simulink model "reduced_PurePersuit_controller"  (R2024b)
settings: Solver=ode1be  StartTime=0.0  StopTime=100  FixedStep=0.01  RelTol=1e-3
undefined symbols (not defined in the file): opti_ref_values, startPose, StepSize, VehicleParams
libraries: slpidlib x1, robotalgslib x1

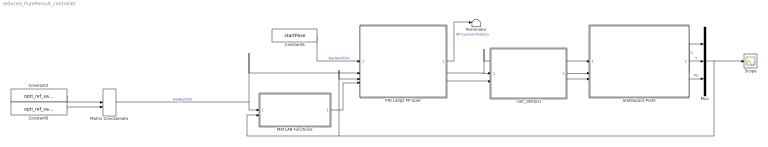
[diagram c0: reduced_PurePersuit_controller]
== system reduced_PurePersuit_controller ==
  Constant2 : Constant  Value=opti_ref_values(:, 1)
  Constant5 : Constant  Value=startPose
  Constant6 : Constant  Value=opti_ref_values(:, 2)
  MATLAB Function2 : MATLAB Function  TreatAsAtomicUnit=on
  Matrix Concatenate : Concatenate  Mode=Multidimensional array  ConcatenateDimension=2
  Mux : Mux  Inputs=3
  PID Längs PP Quer : Subsystem
  Scope : Scope
  StateSpace Plant : Subsystem
  Terminator : Terminator
  calc_delta(s) : Subsystem
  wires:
  Matrix Concatenate/1 -> PID Längs PP Quer/2(Waypoints (HybridAStar)), MATLAB Function2/1(Ref)  "wegpunkte"
  Constant2/1 -> Matrix Concatenate/1
  Constant6/1 -> Matrix Concatenate/2
  Constant5/1 -> PID Längs PP Quer/1(Start Position)  "startposition"
  MATLAB Function2/1(e_long) -> PID Längs PP Quer/4(e_long)
  PID Längs PP Quer/2(v_vehicleBody) -> StateSpace Plant/1(v_vehicleBody), calc_delta(s)/1(vx)
  PID Längs PP Quer/3(Psi_dot) -> calc_delta(s)/2(psi_dot)
  PID Längs PP Quer/1(PP Current Position) -> Terminator/1  "PP Current Position"
  calc_delta(s)/1(delta_f) -> StateSpace Plant/2(Delta_F)
  calc_delta(s)/2(delta_r) -> StateSpace Plant/3(Delta_R)
  StateSpace Plant/1(X) -> Mux/1  "X"
  StateSpace Plant/2(Y) -> Mux/2  "Y"
  StateSpace Plant/3(psi) -> Mux/3  "Psi"
  Mux/1 -> PID Längs PP Quer/3(Current Position), MATLAB Function2/2(Act), Scope/1

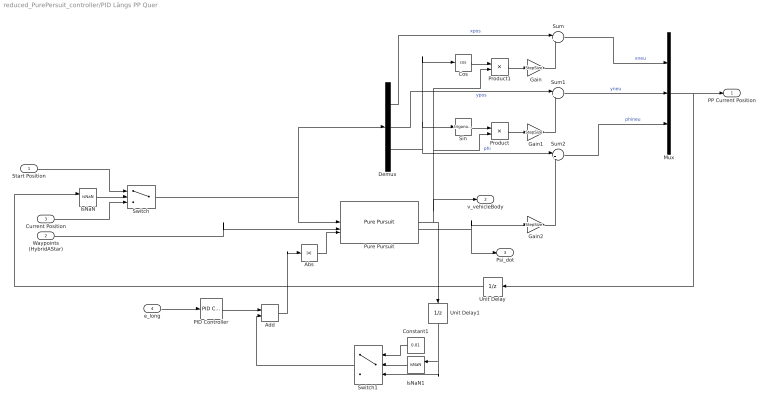
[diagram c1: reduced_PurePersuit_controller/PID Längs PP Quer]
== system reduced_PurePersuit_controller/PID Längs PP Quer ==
  Start Position : Inport
  Waypoints (HybridAStar) : Inport  Port=2
  Current Position : Inport  Port=3
  e_long : Inport  Port=4
  Abs : Abs
  Add : Sum
  Constant1 : Constant  Value=0.01
  Cos : Trigonometry  Operator=cos
  Demux : Demux  Outputs=3
  Gain : Gain  Gain=StepSize
  Gain1 : Gain  Gain=StepSize
  Gain2 : Gain  Gain=StepSize
  IsNaN : RelationalOperator  Operator=isNaN  OutDataTypeStr=boolean  RndMeth=Simplest
  IsNaN1 : RelationalOperator  Operator=isNaN  OutDataTypeStr=boolean  RndMeth=Simplest
  Mux : Mux  Inputs=3
  PID Controller : slpidlib/PID Controller  Controller=PID  Form=Parallel  TimeDomain=Continuous-time  UseExternalTs=off  SampleTime=-1  IntegratorMethod=Forward Euler  FilterMethod=Forward Euler  ControllerParametersSource=internal  P=0.4  I=0  UseKiTs=off  D=0  UseExternalDerivativeSource=off  N=100  UseFilter=on  TunerSelectOption=Transfer Function Based (PID Tuner App)  InitialConditionSource=internal  InitialConditionForIntegrator=0  InitialConditionForFilter=0  DifferentiatorICPrevScaledInput=0  ExternalReset=none  TrackingMode=off  Kt=1  LimitOutput=on  SatLimitsSource=internal  UpperSaturationLimit=1  LowerSaturationLimit=-1  LinearizeAsGain=on  AntiWindupMode=clamping  Kb=1  LimitIntegrator=off  UpperIntegratorSaturationLimit=inf  LowerIntegratorSaturationLimit=-inf  POutMin=[]  POutMax=[]  IOutMin=[]  IOutMax=[]  DOutMin=[]  DOutMax=[]  NOutMin=[]  NOutMax=[]  SumOutMin=[]  SumOutMax=[]  SaturationOutMin=[]  SaturationOutMax=[]  PParamMin=[]  PParamMax=[]  IParamMin=[]  IParamMax=[]  DParamMin=[]  DParamMax=[]  NParamMin=[]  NParamMax=[]  KbParamMin=[]  KbParamMax=[]  KtParamMin=[]  KtParamMax=[]  KbOutMin=[]  KbOutMax=[]  KtOutMin=[]  KtOutMax=[]  IntegratorOutMin=[]  IntegratorOutMax=[]  FilterOutMin=[]  FilterOutMax=[]  SumI1OutMin=[]  SumI1OutMax=[]  SumI2OutMin=[]  SumI2OutMax=[]  SumI3OutMin=[]  SumI3OutMax=[]  SumI4OutMin=[]  SumI4OutMax=[]  SumDOutMin=[]  SumDOutMax=[]  DifferentiatorOutMin=[]  DifferentiatorOutMax=[]  FilterDiffOutCoefMin=[]  FilterDiffOutCoefMax=[]  ReciprocalOutMin=[]  ReciprocalOutMax=[]  SumDenOutMin=[]  SumDenOutMax=[]  SumNumOutMin=[]  SumNumOutMax=[]  DivideOutMin=[]  DivideOutMax=[]  UdiffTsProdOutMin=[]  UdiffTsProdOutMax=[]  NTsProdOutMin=[]  NTsProdOutMax=[]  UintegralTsProdOutMin=[]  UintegralTsProdOutMax=[]  UngainTsProdOutMin=[]  UngainTsProdOutMax=[]  ClampingZeroOutDataTypeStr=Inherit: Inherit via back propagation  ClampingZeroOutMin=[]  ClampingZeroOutMax=[]  FilterDenConstantOutDataTypeStr=Inherit: Inherit via back propagation  FilterDenConstantOutMin=[]  FilterDenConstantOutMax=[]  PCopyOutDataTypeStr=Inherit: Inherit via back propagation  PCopyOutMin=[]  PCopyOutMax=[]  NCopyOutDataTypeStr=Inherit: Inherit via back propagation  NCopyOutMin=[]  NCopyOutMax=[]  IntegratorContinuousStateAttributes=''  IntegratorStateMustResolveToSignalObject=off  IntegratorRTWStateStorageClass=Auto  FilterContinuousStateAttributes=''  FilterStateMustResolveToSignalObject=off  FilterRTWStateStorageClass=Auto  ParallelPVariant=InternalParameters  IdealPVariant=Disabled  IVariant=InternalParameters  DVariant=InternalParameters  IntegratorVariant=Continuous  SatVariant=Enabled  AWVariant=ContClampingParallel  PCopyVariant=Disabled  TRVariant=Disabled  FdbkBlocksVariant=Forward  IdealPFdbkVariant=Disabled  SatFdbkVariant=Disabled  DerivativeFilterVariant=ContFilter  NVariant=InternalParameters  NCopyVariant=Disabled  FilterICVariant=InternalICsFilter  IntegratorICVariant=InternalICs  ExternalResetVariant=Disabled  TRSumVariant=Passthrough  SumFdbkVariant=Disabled  SumVariant=Sum_PID  TsampFilterVariant=InternalTs  TsampNgainVariant=Passthrough  TsampIntegralVariant=Disabled_SignalSpec  ExternalSaturationOutDataTypeStr=Inherit: Same as second input  DerivativeSourceVariant=ErrorSignal  PreIntVariant=InternalPreInt
  Product : Product
  Product1 : Product
  Pure Pursuit : robotalgslib/Pure Pursuit  DesiredLinearVelocityPort=on  DesiredLinearVelocity=v_vb  MaxAngularVelocity=psi_dot_max  LookaheadDistancePort=off  LookaheadDistance=lookahead_distance  TargetDirPort=off  SimulateUsing=Code generation
  Sin : Trigonometry
  Sum : Sum  Inputs=|++
  Sum1 : Sum  Inputs=|++
  Sum2 : Sum  Inputs=|++
  Switch : Switch  Criteria=u2 ~= 0
  Switch1 : Switch  Criteria=u2 ~= 0
  Unit Delay : UnitDelay  SampleTime=-1  HasFrameUpgradeWarning=on
  Unit Delay1 : UnitDelay  SampleTime=-1  HasFrameUpgradeWarning=on
  PP Current Position : Outport
  v_vehicleBody : Outport  Port=2
  Psi_dot : Outport  Port=3
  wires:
  Unit Delay/1 -> IsNaN/1
  Sum/1 -> Mux/1  "xneu"
  Demux/1 -> Sum/1  "xpos"
  Waypoints (HybridAStar)/1 -> Pure Pursuit/2
  Cos/1 -> Product1/1
  Gain2/1 -> Sum2/2
  Pure Pursuit/2 -> Psi_dot/1, Gain2/1
  Gain/1 -> Sum/2
  Sum2/1 -> Mux/3  "phineu"
  Demux/2 -> Sum1/1  "ypos"
  Sin/1 -> Product/1
  Mux/1 -> Unit Delay/1, PP Current Position/1
  Gain1/1 -> Sum1/2
  Product/1 -> Gain1/1
  Sum1/1 -> Mux/2  "yneu"
  IsNaN/1 -> Switch/2
  Start Position/1 -> Switch/1
  Switch/1 -> Demux/1, Pure Pursuit/1
  Demux/3 -> Sum2/1, Sin/1, Cos/1  "phi"
  Product1/1 -> Gain/1
  Current Position/1 -> Switch/3
  Constant1/1 -> Switch1/1
  IsNaN1/1 -> Switch1/2
  Switch1/1 -> Add/2
  e_long/1 -> PID Controller/1
  PID Controller/1 -> Add/1
  Add/1 -> Abs/1
  Pure Pursuit/1 -> Unit Delay1/1, Product/2, Product1/2, v_vehicleBody/1
  Abs/1 -> Pure Pursuit/3
  Unit Delay1/1 -> Switch1/3, IsNaN1/1

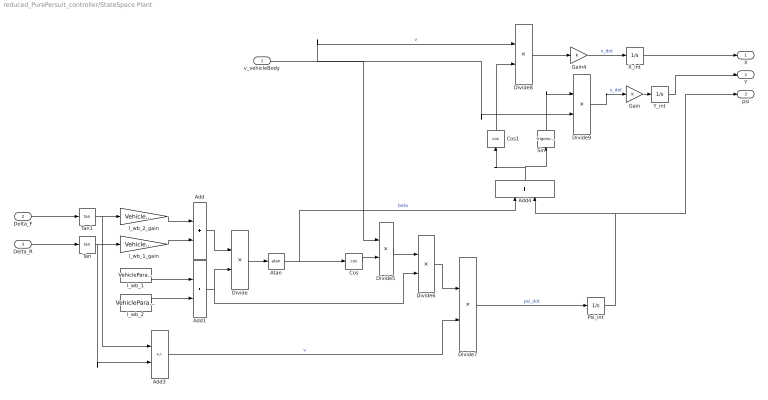
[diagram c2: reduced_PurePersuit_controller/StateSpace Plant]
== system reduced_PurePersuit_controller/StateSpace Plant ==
  v_vehicleBody : Inport
  Delta_F : Inport  Port=2
  Delta_R : Inport  Port=3
  Add : Sum
  Add1 : Sum
  Add3 : Sum  Inputs=+-
  Add4 : Sum
  Atan : Trigonometry  Operator=atan
  Cos : Trigonometry  Operator=cos
  Cos1 : Trigonometry  Operator=cos
  Divide : Product  Inputs=*/
  Divide{5,7..9} (4 alike) : Product  Inputs=**
  Divide6 : Product  Inputs=*/
  Gain : Gain
  Gain4 : Gain
  Psi_int : Integrator
  Sin : Trigonometry
  Tan : Trigonometry  Operator=tan
  Tan1 : Trigonometry  Operator=tan
  X_int : Integrator
  Y_int : Integrator
  l_wb_1 : Constant  Value=VehicleParams.dim_Wheelbase_Road/2
  l_wb_1_gain : Gain  Gain=VehicleParams.dim_Wheelbase_Road/2
  l_wb_2 : Constant  Value=VehicleParams.dim_Wheelbase_Road/2
  l_wb_2_gain : Gain  Gain=VehicleParams.dim_Wheelbase_Road/2
  X : Outport
  Y : Outport  Port=2
  psi : Outport  Port=3
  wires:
  v_vehicleBody/1 -> Divide5/1, Divide9/2, Divide8/1  "v"
  Psi_int/1 -> psi/1, Add4/2
  Add4/1 -> Cos1/1, Sin/1
  Cos1/1 -> Divide8/2
  Sin/1 -> Divide9/1
  Divide8/1 -> Gain4/1
  Divide9/1 -> Gain/1  "y_dot"
  X_int/1 -> X/1
  Y_int/1 -> Y/1
  Gain4/1 -> X_int/1  "x_dot"
  Atan/1 -> Add4/1, Cos/1  "beta"
  Cos/1 -> Divide5/2
  Divide6/1 -> Divide7/1
  l_wb_1_gain/1 -> Add/2
  Add/1 -> Divide/1
  Divide7/1 -> Psi_int/1  "psi_dot"
  Add3/1 -> Divide7/2  "v"
  Add1/1 -> Divide6/2, Divide/2
  Divide5/1 -> Divide6/1
  l_wb_2/1 -> Add1/2
  Divide/1 -> Atan/1
  Tan1/1 -> Add3/1, l_wb_2_gain/1
  l_wb_1/1 -> Add1/1
  Tan/1 -> Add3/2, l_wb_1_gain/1
  l_wb_2_gain/1 -> Add/1
  Gain/1 -> Y_int/1
  Delta_F/1 -> Tan1/1
  Delta_R/1 -> Tan/1

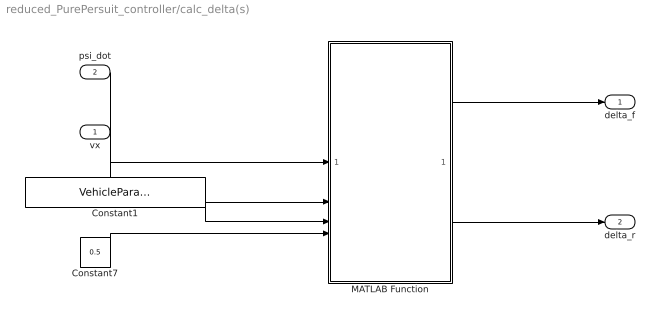
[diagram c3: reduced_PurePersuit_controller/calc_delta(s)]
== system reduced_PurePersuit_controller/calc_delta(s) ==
  vx : Inport
  psi_dot : Inport  Port=2
  Constant1 : Constant  Value=VehicleParams.dim_Wheelbase_Road
  Constant7 : Constant  Value=0.5
  MATLAB Function : MATLAB Function  TreatAsAtomicUnit=on
  delta_f : Outport
  delta_r : Outport  Port=2
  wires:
  vx/1 -> MATLAB Function/2(vx)
  Constant7/1 -> MATLAB Function/4(k)
  Constant1/1 -> MATLAB Function/3(L)
  psi_dot/1 -> MATLAB Function/1(psi_dot)
  MATLAB Function/1(delta_f) -> delta_f/1
  MATLAB Function/2(delta_r) -> delta_r/1

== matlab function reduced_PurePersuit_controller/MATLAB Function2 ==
function e_long = calculate_longitudinal_error(Ref, Act)
    % Berechnet den Längsfehler zwischen einem Referenzpfad und einer echten Position in Echtzeit.
    %
    % Inputs:
    %   X_ref, Y_ref, Psi_ref: Skalare Werte der Referenzposition und -orientierung
    %   X_act, Y_act: Skalare Werte der aktuellen Position
    %
    % Output:
    %   longitudinal_error: Skalarer Wert des berechneten Längsfehlers
    
    X_ref = Ref(1);
    Y_ref = Ref(2);
    Psi_ref = Ref(3);

    X_act = Act(1);
    Y_act = Act(2);
    Psi_act = Act(3);

    % Berechnet den Längsfehler zwischen dem aktuellen Fahrzeugpunkt und dem Referenzpunkt.
    %
    % Eingabe:
    %   X_ref, Y_ref  - Koordinaten des aktuellen Referenzpunktes
    %   Psi_ref       - Orientierung des Referenzpfads am aktuellen Punkt (in Radiant)
    %   X_act, Y_act  - Koordinaten des aktuellen Fahrzeugpunktes
    %
    % Ausgabe:
    %   e_long - Längsfehler (positiv: vor dem Referenzpunkt, negativ: dahinter)

    % Vektor vom Referenzpunkt zum aktuellen Punkt
    dx = X_act - X_ref;
    dy = Y_act - Y_ref;

    % Längsfehler als Projektion des Positionsfehlers auf die Referenzrichtung
    e_long = dx * cos(Psi_ref) + dy * sin(Psi_ref);
end

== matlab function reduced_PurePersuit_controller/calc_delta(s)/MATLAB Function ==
function [delta_f, delta_r] = calculateSteeringAngle(psi_dot, vx, L, k)
    % psi_dot: Giergeschwindigkeit (rad/s)
    % v: Longitudinale Geschwindigkeit (m/s)
    % l: Radstand des Fahrzeugs (m)
    % k: Skalierungsfaktor zur bestimmung der aufteilung der Lenkwinkel (je geringer, desto geringer der Lenkanteil der Hinterräder).
    

    %% Überprüfung, ob Geschwindigkeit > 0 ist
    %if v <= 0
    %    error('Die Geschwindigkeit muss größer als 0 sein.');
    %end

    %% Lenkwinkelberechnung
    %delta_f = atan((l * psi_dot) / v);

    % Lenkwinkelberechnung
    delta_f = atan(k * (L / vx) * psi_dot);
    delta_r = -(atan((1 - k) * (L / vx) * psi_dot));

end
